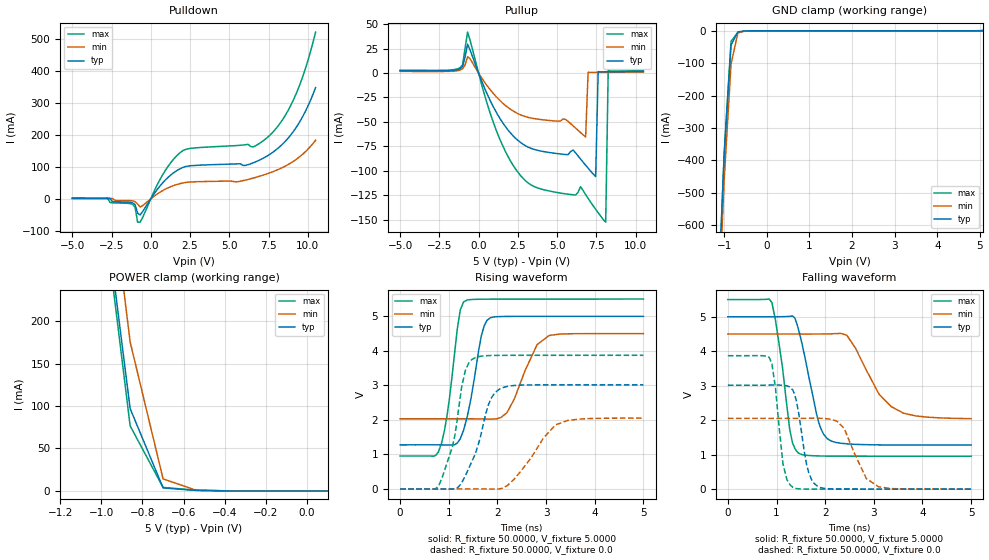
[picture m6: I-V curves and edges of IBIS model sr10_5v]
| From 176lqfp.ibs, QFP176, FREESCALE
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[Model] sr10_5v
|   Model sr10_5v
Model_type 3-state
Polarity   Non-Inverting
Enable   Active-High
Vmeas = 2.5
C_comp   4.6864pF   4.5021pF   4.9391pF
[Temperature Range]   25.0000   0.1500k   -40.0000
[Voltage Range]   5.0000V   4.5000V   5.5000V
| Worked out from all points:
|   slope of the pulldown table from 0 to 0.75 V, typ, clamps not added: 15.2 ohm
|   slope of the pullup table from 0 to 0.75 V, typ, clamps not added: 26.3 ohm
|   GND clamp passes 1 mA (typ) near -0.55 V on its own axis
|   POWER clamp passes 1 mA (typ) near -0.56 V on its own axis
|   rising waveform, R_fixture 50.0000, V_fixture 5.0000: 20-80 % time 281ps typ, 442ps min, 239ps max; typ from 1.28 V to 5 V
|   rising waveform, R_fixture 50.0000, V_fixture 0.0: 20-80 % time 397ps typ, 635ps min, 319ps max; typ from 0 V to 3.02 V
|   falling waveform, R_fixture 50.0000, V_fixture 5.0000: 20-80 % time 333ps typ, 608ps min, 248ps max; typ from 5 V to 1.28 V
|   falling waveform, R_fixture 50.0000, V_fixture 0.0: 20-80 % time 211ps typ, 386ps min, 167ps max; typ from 3.02 V to 0 V
[Pulldown]
|Voltage   I(typ)   I(min)   I(max)
-5V       1.48mA     840uA      2.45mA
-1.16V    -12.51mA   -6.53mA    -17.21mA
-1V       -18.28mA   -8.656mA   -25.93mA
-840mV    -44.65mA   -16.35mA   -72.94mA
-680mV    -50.44mA   -25.63mA   -73.04mA
760mV     49.96mA    25.7mA     75.43mA
2.04V     97.94mA    49.43mA    150.2mA
7V        122.7mA    71.54mA    175.6mA
7.96V     152.3mA    88.21mA    218.4mA
8.92V     199.6mA    111.9mA    292mA
9.72V     260.9mA    141.2mA    387.6mA
10.5V     347.6mA    183mA      520.8mA
[Pullup]
|Voltage   I(typ)   I(min)   I(max)
-5V       2.3mA      1.7mA      2.9mA
-1.18V    4.387mA    3mA        5.364mA
-700mV    29.53mA    16.66mA    41.8mA
900mV     -33.27mA   -20.16mA   -48.58mA
2.34V     -66.41mA   -40.1mA    -97.66mA
6.82V     -94.17mA   -65.35mA   -124.2mA
6.98V     -97.22mA   777uA      -128mA
7.46V     -105.8mA   706uA      -139.2mA
7.62V     1.412mA    720uA      -142.7mA
8.1V      1.252mA    760uA      -152.4mA
8.26V     1.274mA    760uA      2.863mA
10.5V     1.54mA     900uA      2.45mA
[GND_clamp]
|Voltage   I(typ)   I(min)   I(max)
-5V       -15.65A    -15.54A    -15.8A
-1.16V    -883.1mA   -945.9mA   -900.9mA
-1V       -378.6mA   -458.6mA   -378.5mA
-840mV    -44.11mA   -102.9mA   -32.53mA
-680mV    -3.439mA   -6.731mA   -5.118mA
-520mV    -530.1uA   -781.9uA   -565.8uA
-360mV    -4.994uA   -45.89uA   -1.591uA
5.08V     230.9pA    1.498mA    9.384pA
[POWER_clamp]
|Voltage   I(typ)   I(min)   I(max)
-5V       11.12A     11.24A     11.12A
-1.02V    405.3mA    491.3mA    392.9mA
-860mV    97.05mA    175.5mA    76.65mA
-700mV    3.541mA    14.18mA    4.132mA
-540mV    594.7uA    858.4uA    773.9uA
100mV     54.85pA    7.446nA    9.775pA
[Ramp]
| variable   typ   min   max
dV/dt_r  1.8094/0.3973n   1.2306/0.5999n   2.3226/0.3146n
dV/dt_f  2.2324/0.3333n   1.4730/0.5834n   2.7269/0.2439n
R_load = 50.0000
[Rising Waveform]
R_fixture= 50.0000
V_fixture= 5.0000
V_fixture_min= 4.5000
V_fixture_max= 5.5000
|time   V(typ)   V(min)   V(max)
0s        1.277V     2.032V     955.1mV
788.1ps   1.277V     2.032V     1.073V
966.1ps   1.273V     2.033V     2.134V
1.175ns   1.326V     2.033V     4.626V
1.306ns   1.706V     2.033V     5.418V
1.67ns    4.433V     2.028V     5.495V
1.858ns   4.962V     2.024V     5.497V
2.196ns   4.997V     2.209V     5.498V
3.066ns   4.999V     4.447V     5.499V
5ns       5V         4.499V     5.5V
[Rising Waveform]
R_fixture= 50.0000
V_fixture= 0.0
V_fixture_min= 0.0
V_fixture_max= 0.0
|time   V(typ)   V(min)   V(max)
0s        110.1nV    192.8nV    368.1nV
800.6ps   734.7uV    82.7uV     118.7mV
1.079ns   -5.902mV   72.85uV    1.241V
1.209ns   74.57mV    62.21uV    2.387V
1.342ns   386.5mV    196.1uV    3.436V
1.476ns   798.2mV    560.5uV    3.752V
1.813ns   2.431V     -1.621mV   3.862V
2.106ns   2.933V     23.24mV    3.869V
3.195ns   3.015V     1.856V     3.871V
5ns       3.016V     2.051V     3.871V
[Falling Waveform]
R_fixture= 50.0000
V_fixture= 5.0000
V_fixture_min= 4.5000
V_fixture_max= 5.5000
|time   V(typ)   V(min)   V(max)
0s        5V         4.5V       5.5V
905.4ps   4.999V     4.5V       5.411V
1.122ns   5.003V     4.5V       3.535V
1.272ns   5.013V     4.5V       1.732V
1.445ns   4.667V     4.5V       1.053V
1.863ns   1.96V      4.5V       963.8mV
2.04ns    1.467V     4.503V     959.2mV
2.445ns   1.315V     4.464V     956mV
3.359ns   1.282V     2.393V     955.4mV
5ns       1.279V     2.045V     955.2mV
[Falling Waveform]
R_fixture= 50.0000
V_fixture= 0.0
V_fixture_min= 0.0
V_fixture_max= 0.0
|time   V(typ)   V(min)   V(max)
0s        3.016V     2.051V     3.871V
850.6ps   3.018V     2.051V     3.822V
978.6ps   3.02V      2.051V     2.936V
1.132ns   3.014V     2.051V     734mV
1.336ns   2.872V     2.052V     54.52mV
1.62ns    706.4mV    2.055V     3.114mV
1.837ns   90.75mV    2.057V     1.211mV
2.389ns   3.777mV    1.768V     284.2uV
3.095ns   1.099mV    69.5mV     95.21uV
5ns       489.1uV    977.9uV    -18.32uV
